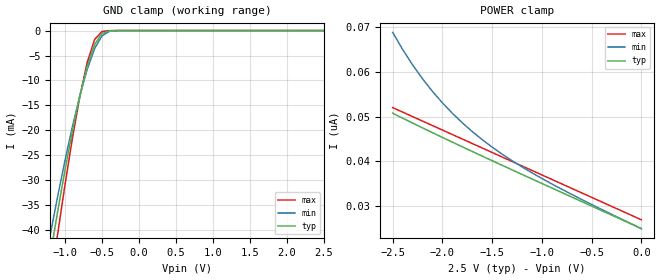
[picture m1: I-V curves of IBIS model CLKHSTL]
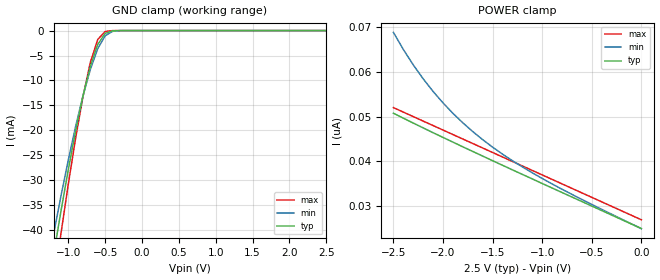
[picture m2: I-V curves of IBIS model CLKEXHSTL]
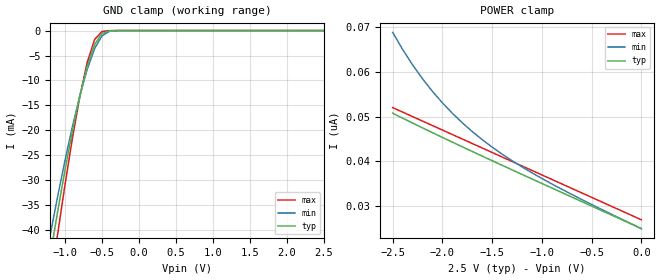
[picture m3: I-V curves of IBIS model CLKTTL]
| IBIS file 72t72105.ibs created by s2ibis2 version 1.1
| North Carolina State University Electronics Research Laboratory  1995
[IBIS ver]   2.1
[File name]   72t72105.ibs
[File Rev]   1.0
[Date]   5/29/01
[Source]   Integrated Device Technology, Inc.
[Notes]   1. Temperatures: typ=25C, min=85C, max=-40C 2. Cemos11.5_2.5v
   process. 3. Ramp rates based on 50 ohm load.
[Copyright]   Copyright 1997, Integrated Device Technology, Inc.
|   Component idt72t72105z
[Component]   idt72t72105z
[Manufacturer]   Integrated Device Technology
[Package]
| variable   typ   min   max
R_pkg   0.75   0.60   0.90
L_pkg   8.50nH   8.30nH   9.90nH
C_pkg   0.53pF   0.46pF   0.60pF
| Note: The following lists pins and their corresponding models based on
|   application.
|   The model_name is obvious and self-explanatory.
|   Please select the models accordingly.
|[Pin]  signal_name   model_name   R_pin   L_pin   C_pin
|   Dx(D0,...)   DATAHSTL/DATAEXHSTL/DATATTL
|   GND   GND
|   WENL   CTRLHSTL/CTRLEXHSTL/CTRLTTL
|   WCSL   CTRLHSTL/CTRLEXHSTL/CTRLTTL
|   WCLK   CLKHSTL/CLKEXHSTL/CLKTTL
|   PRSL   CTRLHSTL/CTRLEXHSTL/CTRLTTL
|   MRSL   CTRLHSTL/CTRLEXHSTL/CTRLTTL
|   LDL   CTRLHSTL/CTRLEXHSTL/CTRLTTL
|   FWFTSI   CTRLHSTL/CTRLEXHSTL/CTRLTTL
|   FFL   FPADHSTL/FPADEXHSTL/FPADTTL
|   PAFL   FPADHSTL/FPADEXHSTL/FPADTTL
|   OW   DATATTL
|   FSEL0   DATATTL
|   HFL   FPADHSTL/FPADEXHSTL/FPADTTL
|   SHSTL   DATATTL
|   FSEL1   DATATTL
|   BEL   DATATTL
|   VDDQ   POWER
|   IP   DATATTL
|   BM   DATATTL
|   RHSTL   DATATTL
|   ASYRL   DATATTL
|   VCC   POWER
|   PAEL   FPADHSTL/FPADEXHSTL/FPADTTL
|   PFM   DATATTL
|   EFL   FPADHSTL/FPADEXHSTL/FPADTTL
|   ERENL   QPADHSTL/QPADEXHSTL/QPADTTL
|   MARK   CTRLHSTL/CTRLEXHSTL/CTRLTTL
|   RCLK   CLKHSTL/CLKEXHSTL/CLKTTL
|   RENL   CTRLHSTL/CTRLEXHSTL/CTRLTTL
|   TRL   CTRLHSTL/CTRLEXHSTL/CTRLTTL
|   RCSL   CTRLHSTL/CTRLEXHSTL/CTRLTTL
|   OEL   CTRLHSTL/CTRLEXHSTL/CTRLTTL
|   Qx(Q0,...)   QPADHSTL/QPADEXHSTL/QPADTTL
|   ERCLK   QPADHSTL/QPADEXHSTL/QPADTTL
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[Pin]  signal_name   model_name   R_pin   L_pin   C_pin
1   DATAHSTL   DATAHSTL
2   DATAEXHSTL   DATAEXHSTL
3   DATATTL   DATATTL
4   CTRLHSTL   CTRLHSTL
5   CTRLEXHSTL   CTRLEXHSTL
6   CTRLTTL   CTRLTTL
7   CLKHSTL   CLKHSTL
8   CLKEXHSTL   CLKEXHSTL
9   CLKTTL   CLKTTL
10   VCC   POWER
11   GND   GND
12   FPADHSTL   FPADHSTL
13   FPADEXHSTL   FPADEXHSTL
14   FPADTTL   FPADTTL
15   VDDQ   POWER
16   QPADHSTL   QPADHSTL
17   QPADEXHSTL   QPADEXHSTL
18   QPADTTL   QPADTTL
19   PUHSTL   PUHSTL
20   PUEXHSTL   PUEXHSTL
21   PUTTL   PUTTL
| Models and submodels in the file (18): CLKHSTL (Input), CTRLHSTL (Input), DATAHSTL (Input), PUHSTL (Input), CLKEXHSTL (Input), CTRLEXHSTL (Input), DATAEXHSTL (Input), PUEXHSTL (Input), CLKTTL (Input), CTRLTTL (Input), DATATTL (Input), PUTTL (Input), QPADEXHSTL (3-state), FPADEXHSTL (3-state), QPADHSTL (3-state), FPADHSTL (3-state), QPADTTL (3-state), FPADTTL (3-state)
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| FIN  FIN   dummy_model
| QIN  QIN   dummy_model
| QOE  QOE   dummy_model
| FOEL FOE   dummy_model
|   Model CLKHSTL
[Model]   CLKHSTL
Model_type   Input
Vinl =  0.250V
Vinh =  1.250V
|Vmeas =  0.750V
C_comp   3.00pF   NA   NA
[Temperature Range]   25.00   85.00   -40.00
[Voltage Range]   2.50V   2.30V   2.70V
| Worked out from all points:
|   GND clamp passes 1 mA (typ) near -0.52 V on its own axis
[GND_clamp]
| voltage   I(typ)   I(min)   I(max)
-2.5V     -171mA     -153mA     -195mA
-1.2V     -45.09mA   -40.91mA   -51.2mA
-1.1V     -36.28mA   -33.25mA   -40.8mA
-1V       -27.91mA   -25.98mA   -30.84mA
-900mV    -20.11mA   -19.21mA   -21.55mA
-800mV    -13.1mA    -13.07mA   -13.22mA
-700mV    -7.177mA   -7.773mA   -6.35mA
-600mV    -2.805mA   -3.616mA   -1.783mA
-500mV    -572uA     -1.059mA   -188uA
-400mV    -51.64uA   -157uA     -8.193uA
-300mV    -2.315uA   -13.07uA   -122nA
2.5V      25.05nA    27.16nA    25nA
[POWER_clamp]
| voltage   I(typ)   I(min)   I(max)
-2.5V     50.75nA    68.77nA    52nA
-2.4V     49.65nA    64.96nA    51nA
-2.3V     48.56nA    61.53nA    50nA
-2.2V     47.48nA    58.42nA    49nA
-2.1V     46.41nA    55.61nA    48nA
-1.9V     44.31nA    50.73nA    46nA
-1.8V     43.26nA    48.61nA    45nA
-1.6V     41.2nA     44.86nA    43nA
-1.3V     38.13nA    40.17nA    40nA
-1V       35.09nA    36.21nA    37nA
-600mV    31.07nA    31.53nA    33nA
0V        25.05nA    25.02nA    27nA
|   Model CLKEXHSTL
[Model]   CLKEXHSTL
Model_type   Input
Vinl =  0.400V
Vinh =  1.400V
|Vmeas =  0.900V
C_comp   3.00pF   NA   NA
[Temperature Range]   25.00   85.00   -40.00
[Voltage Range]   2.50V   2.30V   2.70V
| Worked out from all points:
|   GND clamp passes 1 mA (typ) near -0.52 V on its own axis
[GND_clamp]
| voltage   I(typ)   I(min)   I(max)
-2.5V     -171mA     -153mA     -195mA
-1.2V     -45.09mA   -40.91mA   -51.2mA
-1.1V     -36.28mA   -33.25mA   -40.8mA
-1V       -27.91mA   -25.98mA   -30.84mA
-900mV    -20.11mA   -19.21mA   -21.55mA
-800mV    -13.1mA    -13.07mA   -13.22mA
-700mV    -7.177mA   -7.773mA   -6.35mA
-600mV    -2.805mA   -3.616mA   -1.783mA
-500mV    -572uA     -1.059mA   -188uA
-400mV    -51.64uA   -157uA     -8.193uA
-300mV    -2.315uA   -13.07uA   -122nA
2.5V      25.05nA    27.16nA    25nA
[POWER_clamp]
| voltage   I(typ)   I(min)   I(max)
-2.5V     50.75nA    68.77nA    52nA
-2.4V     49.65nA    64.96nA    51nA
-2.3V     48.56nA    61.53nA    50nA
-2.2V     47.48nA    58.42nA    49nA
-2.1V     46.41nA    55.61nA    48nA
-1.9V     44.31nA    50.73nA    46nA
-1.8V     43.26nA    48.61nA    45nA
-1.6V     41.2nA     44.86nA    43nA
-1.3V     38.13nA    40.17nA    40nA
-1V       35.09nA    36.21nA    37nA
-600mV    31.07nA    31.53nA    33nA
0V        25.05nA    25.02nA    27nA
|   Model CLKTTL
[Model]   CLKTTL
Model_type   Input
Vinl =  0.000V
Vinh =  2.500V
|Vmeas =  1.250V
C_comp   3.00pF   NA   NA
[Temperature Range]   25.00   85.00   -40.00
[Voltage Range]   2.50V   2.30V   2.70V
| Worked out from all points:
|   GND clamp passes 1 mA (typ) near -0.52 V on its own axis
[GND_clamp]
| voltage   I(typ)   I(min)   I(max)
-2.5V     -171mA     -153mA     -195mA
-1.2V     -45.09mA   -40.91mA   -51.2mA
-1.1V     -36.28mA   -33.25mA   -40.8mA
-1V       -27.91mA   -25.98mA   -30.84mA
-900mV    -20.11mA   -19.21mA   -21.55mA
-800mV    -13.1mA    -13.07mA   -13.22mA
-700mV    -7.177mA   -7.773mA   -6.35mA
-600mV    -2.805mA   -3.616mA   -1.783mA
-500mV    -572uA     -1.059mA   -188uA
-400mV    -51.64uA   -157uA     -8.193uA
-300mV    -2.315uA   -13.07uA   -122nA
2.5V      25.05nA    27.16nA    25nA
[POWER_clamp]
| voltage   I(typ)   I(min)   I(max)
-2.5V     50.75nA    68.77nA    52nA
-2.4V     49.65nA    64.96nA    51nA
-2.3V     48.56nA    61.53nA    50nA
-2.2V     47.48nA    58.42nA    49nA
-2.1V     46.41nA    55.61nA    48nA
-1.9V     44.31nA    50.73nA    46nA
-1.8V     43.26nA    48.61nA    45nA
-1.6V     41.2nA     44.86nA    43nA
-1.3V     38.13nA    40.17nA    40nA
-1V       35.09nA    36.21nA    37nA
-600mV    31.07nA    31.53nA    33nA
0V        25.05nA    25.02nA    27nA
